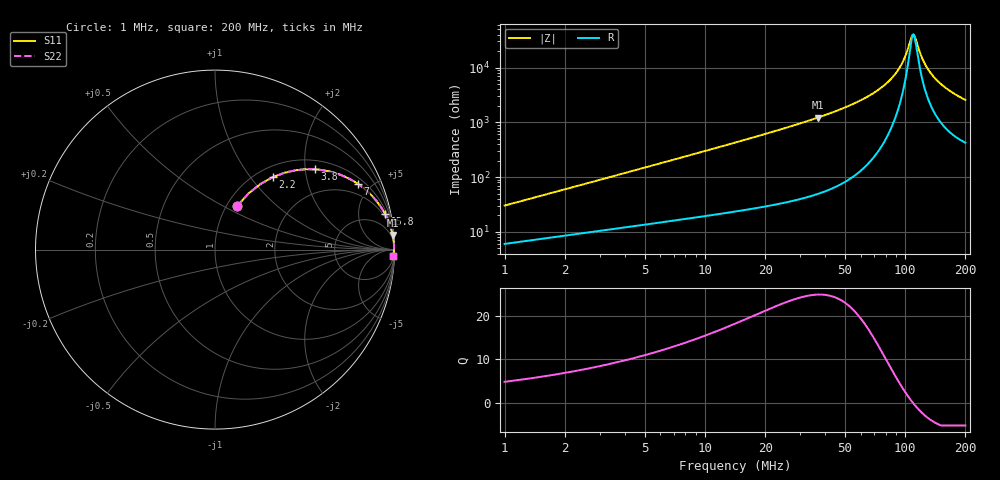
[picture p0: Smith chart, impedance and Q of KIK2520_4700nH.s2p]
!version-2
!date-01.2022
!Series
# MHz S RI R 50
!Freq ReS11 ImS11 ReS21 ImS21 ReS12 ImS12 ReS22 ImS22
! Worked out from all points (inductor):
!   499 points, 1 MHz to 200 MHz, reference 50 ohm
!   read as one part in series: L = 4.69 uH near 1.8 MHz
!   highest Q = 24.8 at 36.6 MHz (marker M1), where L = 5.28 uH
!   self-resonance near 109.8 MHz
!   S11 on the Smith chart (normalised r, x): 1 MHz: 1.12, +0.59; 2.2 MHz: 1.18, +1.30; 3.8 MHz: 1.23, +2.24; 7 MHz: 1.32, +4.15; 15.8 MHz: 1.50, +9.52; 200 MHz: 9, -51
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1  0.1244 0.2437  0.8756 -0.2437  0.8756 -0.2437  0.1244 0.2437
2.2  0.3226 0.4039  0.6774 -0.4039  0.6774 -0.4039  0.3226 0.4039
3.8  0.5545 0.4475  0.4455 -0.4475  0.4455 -0.4475  0.5545 0.4475
5.4  0.7038 0.4148  0.2962 -0.4148  0.2962 -0.4148  0.7038 0.4148
7  0.7945 0.3673  0.2055 -0.3673  0.2055 -0.3673  0.7945 0.3673
10.6  0.8948 0.2769  0.1052 -0.2769  0.1052 -0.2769  0.8948 0.2769
15.8  0.9484 0.1966  0.0516 -0.1966  0.0516 -0.1966  0.9484 0.1966
23.8  0.9763 0.1315  0.0237 -0.1315  0.0237 -0.1315  0.9763 0.1315
34.2  0.9885 0.0881  0.0115 -0.0881  0.0115 -0.0881  0.9885 0.0881
36.6  0.99 0.0812  0.00996 -0.0812  0.00996 -0.0812  0.99 0.0812
67.4  0.9971 0.0312  0.00293 -0.0312  0.00293 -0.0312  0.9971 0.0312
87.8  0.9978 0.0139  0.00224 -0.0139  0.00224 -0.0139  0.9978 0.0139
95  0.9978 0.00903  0.00224 -0.00903  0.00224 -0.00903  0.9978 0.00903
100.6  0.9977 0.0055  0.00229 -0.0055  0.00229 -0.0055  0.9977 0.0055
107.8  0.9976 0.00127  0.00243 -0.00127  0.00243 -0.00127  0.9976 0.00127
110.2  0.9975 -7.44e-05  0.00249 7.44e-05  0.00249 7.44e-05  0.9975 -7.44e-05
112.2  0.9975 -0.00117  0.00255 0.00117  0.00255 0.00117  0.9975 -0.00117
122.2  0.9971 -0.00638  0.00288 0.00638  0.00288 0.00638  0.9971 -0.00638
133.8  0.9966 -0.012  0.00338 0.012  0.00338 0.012  0.9966 -0.012
148.2  0.9959 -0.0183  0.00413 0.0183  0.00413 0.0183  0.9959 -0.0183
167  0.9947 -0.0259  0.00532 0.0259  0.00532 0.0259  0.9947 -0.0259
200  0.9921 -0.038  0.00787 0.038  0.00787 0.038  0.9921 -0.038
